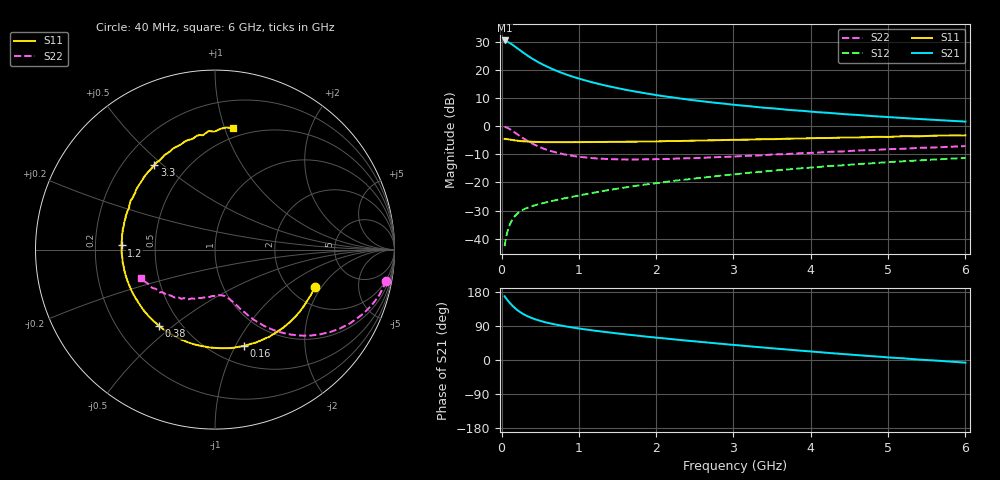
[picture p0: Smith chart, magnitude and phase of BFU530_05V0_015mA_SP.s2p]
! Filename:  P:\Prog\Test\Noise\ATS_data\Testdata_Net\03 Spar\BFU530_APG2013_40_A05_05p0V_015mA_SP_CM01_D.s2p
! Date/Time: Fri 26/Apr/2013 13:03:15
! BFU530_APG2013_40_A05_05p0V_1to25mA_SP_CM01_Bias6_R.s2p
! MDIF S-parameter v. bias file
! BFU530_APG2013_40_A05_05p0V_1to25mA_SP_CM01
! Date/time Wed Apr 24 19:36:53 2013
! VAR V_out= 5.0000
! VAR I_out= 15.0000
! VAR V_in= 0.8357
! VAR I_in= 0.1660
! Device data file deembeded for feedlines and parallel
! Original file: \03 Spar\BFU530_APG2013_40_A05_05p0V_015mA_SP_CM01_R.s2p
! Feed-files: PR047V01_250413_Feed1.s2p, PR047V01_250413_Feed2.s2p
! Parallel-file: PR047V01_250413_Par.s2p
# MHz S MA R 50
!  Freq-MHz  S11-mag  S11-arg  S21-mag  S21-arg  S12-mag  S12-arg  S22-mag  S22-arg
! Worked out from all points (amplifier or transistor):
!   98 points, 40 MHz to 6 GHz, reference 50 ohm
!   highest |S21| = 30.4 dB at 40 MHz (marker M1)
!   |S21| within 3 dB of that: start of sweep to 215.9 MHz
!   unconditionally stable (mu >= 1): 1.474 GHz to 3.756 GHz
!   at 300 MHz: K = 0.40, MSG = 27.6 dB, |S12| = -29.4 dB
!   at 1.6 GHz: K = 1.02, MAG = 16.5 dB, |S12| = -21.8 dB
!   at 6 GHz: K = 0.87, MSG = 6.5 dB, |S12| = -11.3 dB
!   S11 on the Smith chart (normalised r, x): 40 MHz: 2.68, -1.74; 160 MHz: 0.69, -1.08; 380 MHz: 0.38, -0.45; 1.2 GHz: 0.31, +0.02; 3.3 GHz: 0.33, +0.47; 6 GHz: 0.42, +1.07
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40  0.5939 -20.6  33.17 168.1  0.007357 81.2  0.9694 -10.3
50  0.5907 -25.7  32.99 164.8  0.009044 79.2  0.9604 -12.8
100  0.5778 -49.2  30.27 152.5  0.01684 70.2  0.8909 -24.4
120  0.572 -58.0  29.2 147.7  0.01947 67.1  0.8576 -28.6
160  0.5601 -73.4  26.68 139.6  0.02396 61.8  0.7889 -35.6
220  0.5465 -92.7  23.27 129.4  0.029 56.2  0.6905 -44.0
260  0.5403 -103.2  21.18 123.9  0.03156 53.7  0.6335 -48.3
320  0.5321 -115.9  18.53 117.1  0.03468 51.0  0.5622 -53.4
380  0.5272 -126.2  16.32 111.7  0.03718 49.6  0.5041 -57.3
440  0.5233 -134.4  14.55 107.2  0.03949 48.9  0.4581 -60.2
500  0.5211 -141.3  13.09 103.4  0.04158 48.6  0.4215 -62.7
650  0.5183 -154.7  10.42 95.7  0.04657 49.2  0.3567 -67.1
850  0.5184 -167.0  8.138 88.0  0.05329 50.8  0.3068 -71.2
1050  0.5193 -176.7  6.664 81.7  0.06032 52.3  0.2806 -74.9
1200  0.5212 177.4  5.859 77.5  0.06579 53.2  0.2684 -77.4
1600  0.5263 164.3  4.426 67.7  0.08109 54.4  0.2558 -84.2
2050  0.5364 153.1  3.467 58.1  0.09866 54.3  0.2589 -92.3
3100  0.5714 129.5  2.32 38.1  0.143 51.0  0.2927 -111.2
3300  0.581 125.5  2.183 34.4  0.152 49.9  0.2997 -114.7
4100  0.6125 110.8  1.762 20.9  0.1875 44.6  0.3382 -128.4
5200  0.6615 93.0  1.389 4.4  0.2371 36.0  0.3948 -146.3
6000  0.6829 81.7  1.201 -7.0  0.2715 28.7  0.4412 -158.7
